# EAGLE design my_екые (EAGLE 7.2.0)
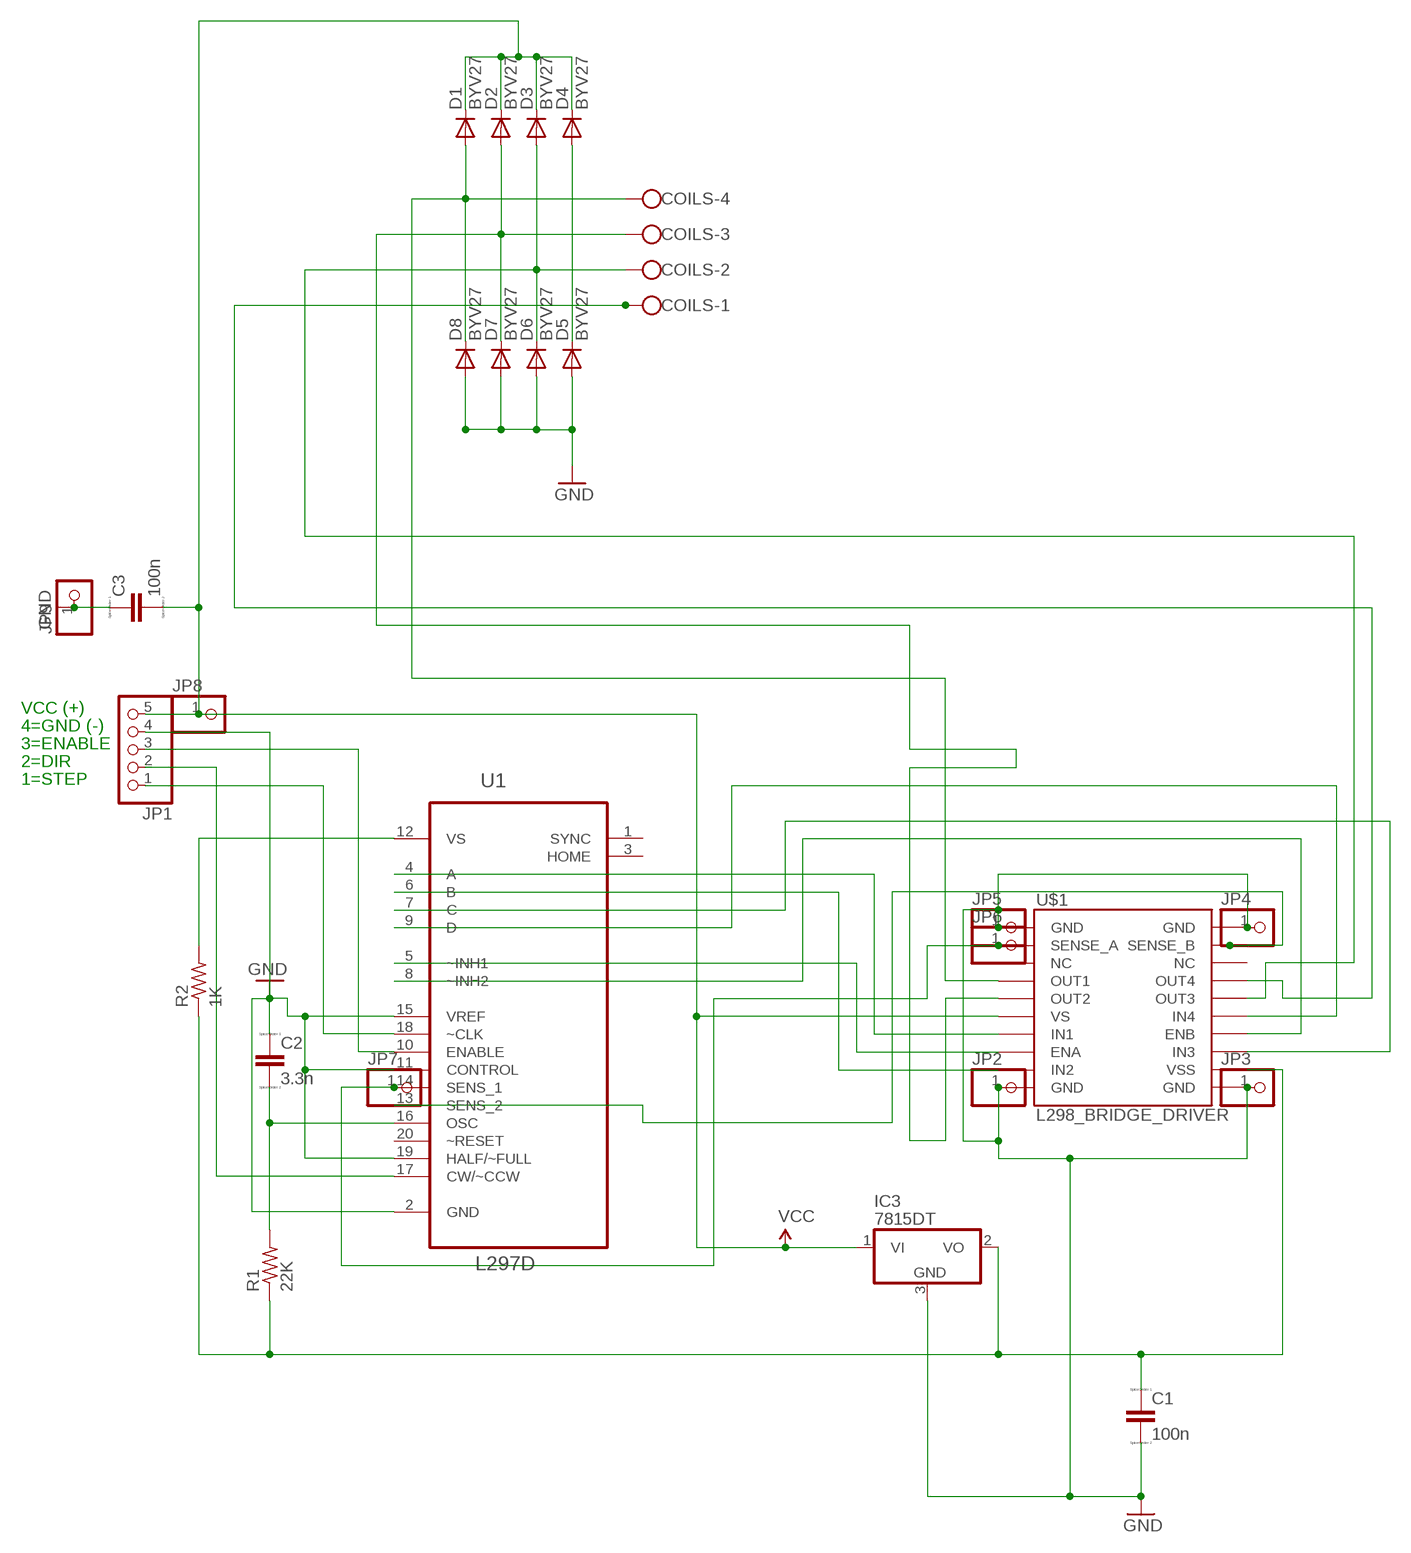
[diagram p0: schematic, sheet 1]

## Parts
C1  100n  CC1206  [C1206]
C2  3.3n  CC1206  [C1206]
C3  100n  CC1206  [C1206]
COILS  W237-4  [W237-4]
D1  BYV27  [SOD57-10]
D2  BYV27  [SOD57-10]
D3  BYV27  [SOD57-10]
D4  BYV27  [SOD57-10]
D5  BYV27  [SOD57-10]
D6  BYV27  [SOD57-10]
D7  BYV27  [SOD57-10]
D8  BYV27  [SOD57-10]
IC3  7815DT  [TO252]
JP1  PINHD-1X55X2MM  [1_05X2MM]
JP2  PINHD-1X1  [1X01]
JP3  PINHD-1X1  [1X01]
JP4  PINHD-1X1  [1X01]
JP5  PINHD-1X1  [1X01]
JP6  PINHD-1X1  [1X01]
JP7  PINHD-1X1  [1X01]
JP8  PINHD-1X1  [1X01]
JP9  PINHD-1X1  [1X01]
R1  22K  RES-US1206  [R1206]
R2  1K  RES-US1206  [R1206]
U1  L297D  [SOIC127P1032X265-20N]
U$1  L298_BRIDGE_DRIVER  [POWERSO20]

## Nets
GND: C1.2 C2.1 C3.1 D5.A D6.A D7.A D8.A IC3.3(GND) JP1.4 JP2.1 JP3.1 JP4.1 JP5.1 JP9.1 U1.2(GND) U1.11(CONTROL) U1.15(VREF) U1.19(HALF/~FULL) U$1.1(GND) U$1.10(GND) U$1.11(GND) U$1.20(GND)
N$1: C1.1 IC3.2(VO) R1.1 R2.1 U$1.12(VSS)
N$2: C2.2 R1.2 U1.16(OSC)
N$3: U1.4(A) U$1.7(IN1)
N$4: U1.6(B) U$1.9(IN2)
N$5: U1.7(C) U$1.13(IN3)
N$6: U1.9(D) U$1.15(IN4)
N$7: U1.5(~INH1) U$1.8(ENA)
N$8: U1.8(~INH2) U$1.14(ENB)
N$9: COILS.4 D1.A D8.C U$1.4(OUT1)
N$10: COILS.3 D2.A D7.C U$1.5(OUT2)
N$11: COILS.2 D3.A D6.C U$1.16(OUT3)
N$12: COILS.1 D4.A D5.C U$1.17(OUT4)
N$13: JP1.1 U1.18(~CLK)
N$14: JP1.3 U1.10(ENABLE)
N$16: JP6.1 JP7.1 U1.14(SENS_1) U$1.2(SENSE_A)
N$17: U1.13(SENS_2) U$1.19(SENSE_B)
N$18: JP1.2 U1.17(CW/~CCW)
N$25: R2.2 U1.12(VS)
VCC: C3.2 D1.C D2.C D3.C D4.C IC3.1(VI) JP1.5 JP8.1 U$1.6(VS)
Unconnected: U1.1(SYNC) U1.3(HOME) U1.20(~RESET) U$1.3(NC) U$1.18(NC)

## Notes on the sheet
- VCC (+)
- 4=GND (-)
- 3=ENABLE
- 2=DIR
- 1=STEP

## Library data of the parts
C1-C3 = eagle-ltspice:C: CAPACITOR, European symbol; SPICEMODEL: NONE; SPICEPREFIX: C
COILS = con-wago-500:W237-4: WAGO SCREW CLAMP
D1-D8 = diode:BYV27: DIODE
IC3 = linear:78*: Positive VOLTAGE REGULATOR Source: http://cache.national.com/ds/LM/LM78L05.pdf http://www.fairchildsemi.com/ds/LM/LM7805.pdf
JP1 = pinhead:PINHD-1X5: PIN HEADER
JP2-JP9 = pinhead:PINHD-1X1: PIN HEADER
R1 R2 = fab:RES-US: Resistor (US Symbol)
U1 = ST Microelctronics_By_element14_Batch_1:L297D: STEPPER MOTOR CONTROLLERS; MPN: L297D; OC_FARNELL: 1467714; OC_NEWARK: 89K0738; PACKAGE: SOICW-20; SUPPLIER: STMICROELECTRONICS
U$1 = SparkFun-PowerIC:L298_BRIDGE_DRIVER: Full-bridge power driver IC

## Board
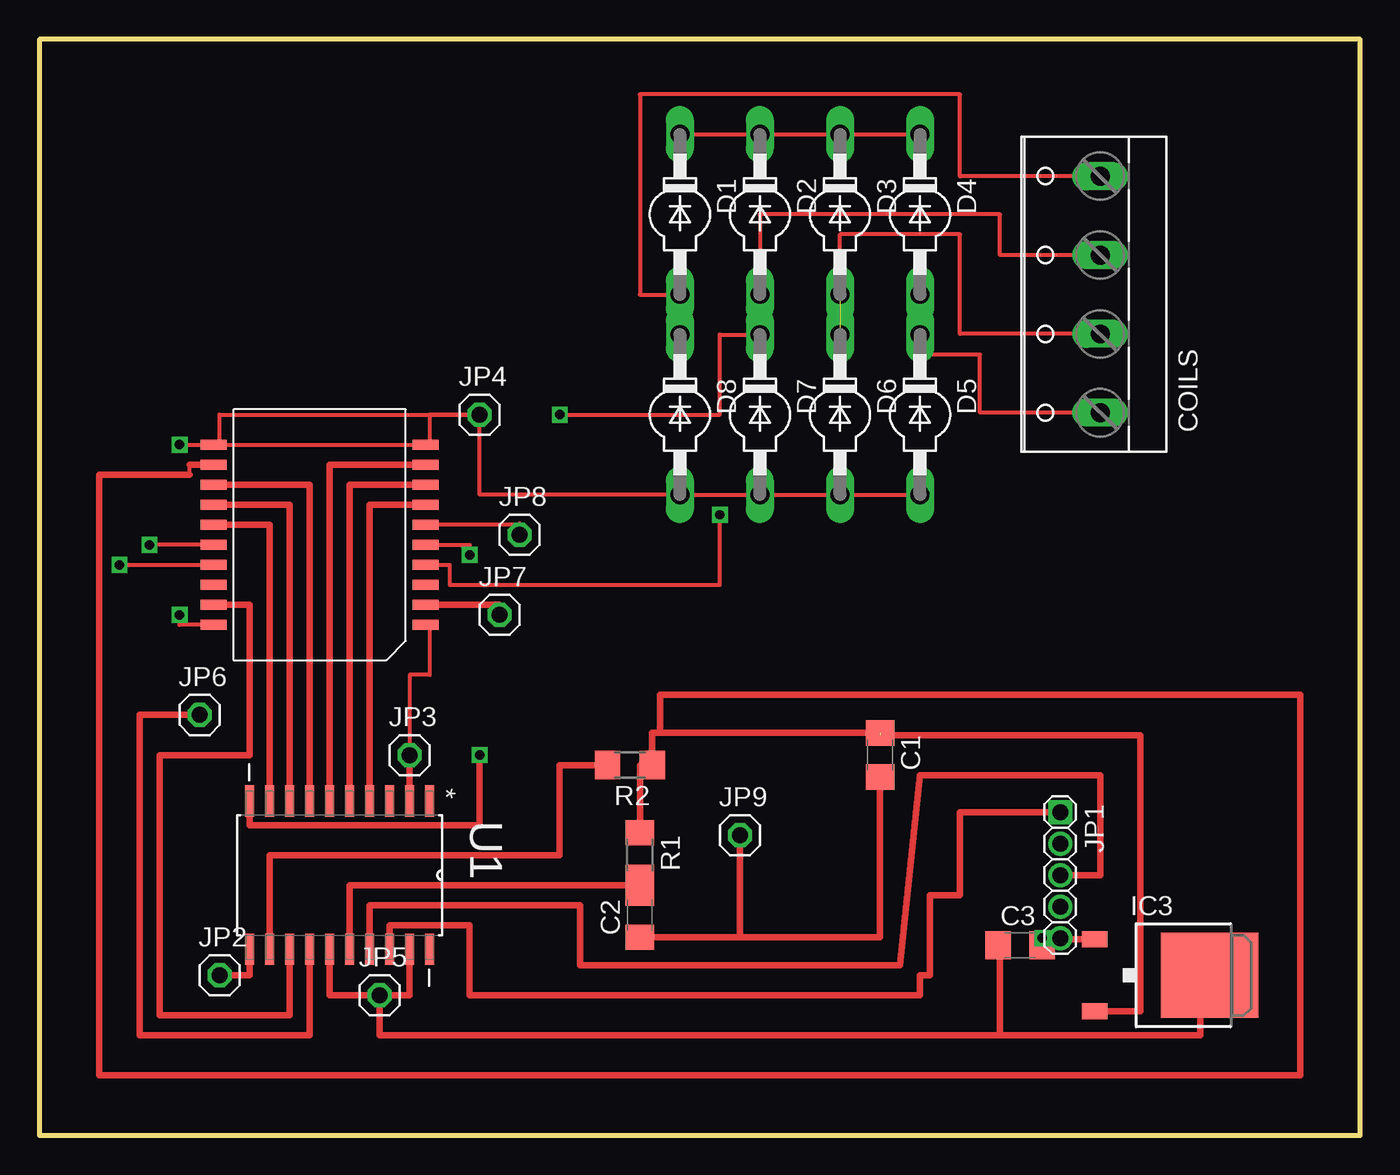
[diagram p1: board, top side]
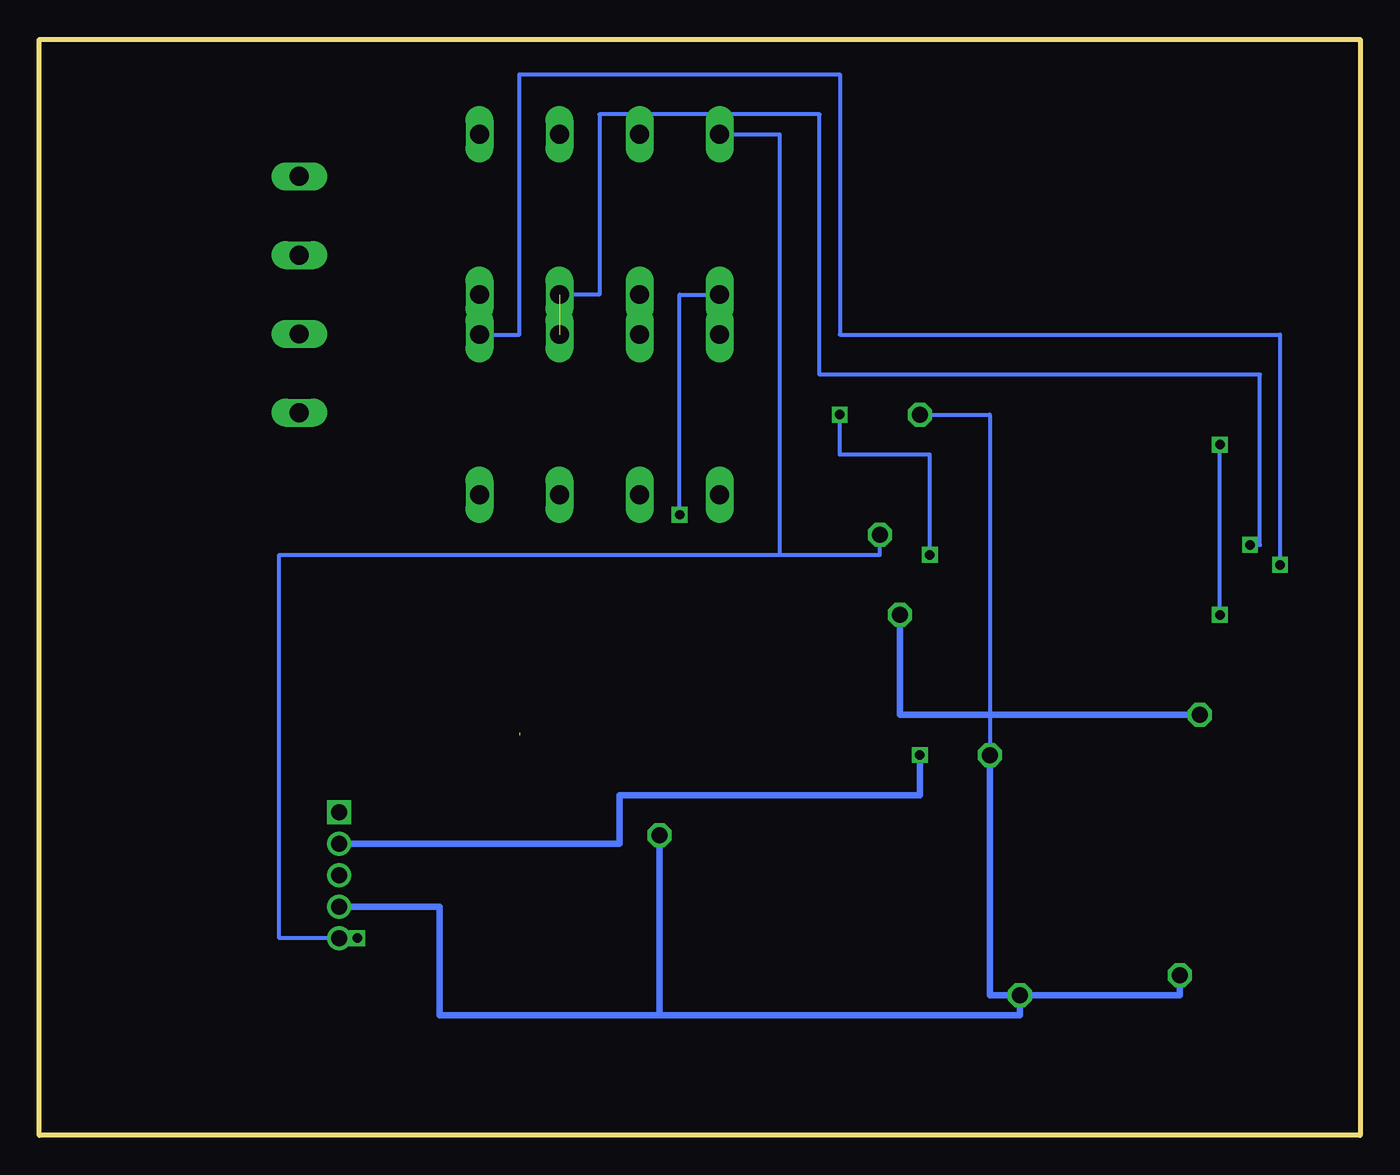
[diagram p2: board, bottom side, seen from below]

Size 83.8 x 69.52 mm. Coordinates in mm from the lower left corner, seen from the top.
Outline: 0,0 83.8,0 83.8,69.52 0,69.52 0,0
Copper layers (1*16): Top 0.035mm / dielectric 1.5mm / Bottom 0.035mm
Design rules "default": minimum track width 10mil, minimum drill 24mil, track to track 8mil, track to pad 8mil, pad to pad 8mil, via to via 8mil, smd to smd 8mil, copper to edge 40mil, drill to drill 8mil, minimum pad ring 10mil, minimum via ring 8mil, stop-mask expansion 4mil, vias tented up to drill 0mil, thermal gap 10mil

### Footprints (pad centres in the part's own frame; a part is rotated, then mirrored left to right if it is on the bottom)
C1206 = smd 1.6 x 1.8: 1 -1.4,0; 2 1.4,0
W237-4 = drill 1.194 long: 1 -7.5,-1.27; 2 -2.5,-1.27; 3 2.5,-1.27; 4 7.5,-1.27
SOD57-10 = drill 1.194 long: A 5.08,0; C -5.08,0
TO252 = smd 1 x 1.6: 1 -2.28,-4.8; 2 2.28,-4.8 | smd 5.4 x 6.2: 3 0,2.5
1_05X2MM = drill 1.016 pad 1.3 square: 1 -4,0 | drill 1.016 pad 1.3: 2 0,0; 3 -2,0; 4 2,0; 5 4,0
1X01 = drill 1.016 octagon: 1 0,0
R1206 = smd 1.6 x 1.803: 1 -1.422,0; 2 1.422,0
SOIC127P1032X265-20N = smd 1.981 x 0.559: 1 -4.699,5.715; 2 -4.699,4.445; 3 -4.699,3.175; 4 -4.699,1.905; 5 -4.699,0.635; 6 -4.699,-0.635; 7 -4.699,-1.905; 8 -4.699,-3.175; 9 -4.699,-4.445; 10 -4.699,-5.715; 11 4.699,-5.715; 12 4.699,-4.445; 13 4.699,-3.175; 14 4.699,-1.905; 15 4.699,-0.635; 16 4.699,0.635; 17 4.699,1.905; 18 4.699,3.175; 19 4.699,4.445; 20 4.699,5.715
POWERSO20 = smd 1.651 x 0.635: 1 -6.731,5.715; 2 -6.731,4.445; 3 -6.731,3.175; 4 -6.731,1.905; 5 -6.731,0.635; 6 -6.731,-0.635; 7 -6.731,-1.905; 8 -6.731,-3.175; 9 -6.731,-4.445; 10 -6.731,-5.715; 11 6.731,-5.715; 12 6.731,-4.445; 13 6.731,-3.175; 14 6.731,-1.905; 15 6.731,-0.635; 16 6.731,0.635; 17 6.731,1.905; 18 6.731,3.175; 19 6.731,4.445; 20 6.731,5.715

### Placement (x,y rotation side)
C1  53.34,24.13 270 top
C2  38.1,13.97 90 top
C3  62.23,12.06 0 top
COILS  66.04,53.34 90 top
D1  40.64,58.42 270 top
D2  45.72,58.42 270 top
D3  50.8,58.42 270 top
D4  55.88,58.42 270 top
D5  55.88,45.72 270 top
D6  50.8,45.72 270 top
D7  45.72,45.72 270 top
D8  40.64,45.72 270 top
IC3  71.75,10.16 270 top
JP1  64.77,16.51 270 top
JP2  11.43,10.16 0 top
JP3  23.5,24.13 0 top
JP4  27.94,45.72 0 top
JP5  21.59,8.89 0 top
JP6  10.16,26.67 0 top
JP7  29.21,33.02 0 top
JP8  30.48,38.1 0 top
JP9  44.45,19.05 0 top
R1  38.1,17.78 270 top
R2  37.46,23.49 180 top
U1  19.05,16.51 270 top
U$1  17.78,38.1 180 top

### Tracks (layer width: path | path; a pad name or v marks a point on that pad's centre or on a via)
GND  (via drill 0.6)
  Top 0.254: 11.43,43.81 U$1.10 | 11.43,43.81 U$1.11 v8.89,43.81 | U$1.20 8.89,32.38 v8.89,33.02 | 11.43,43.81 11.43,45.72 JP4.1 | JP4.1 24.76,45.72 24.76,43.81 | U$1.1 24.76,32.38 24.76,29.21 23.5,29.21 JP3.1 | D5.A D6.A D7.A D8.A 27.94,40.64 JP4.1
  Top 0.406: JP2.1 13.33,10.16 U1.11 | U1.19 23.5,8.89 JP5.1 | JP5.1 18.42,8.89 U1.15 | U1.2 JP3.1 | C2.1 44.45,12.57 | C1.2 53.34,12.57 44.45,12.57 | C3.1 60.96,12.06 60.96,6.35 | 60.96,6.35 21.59,6.35 JP5.1 | IC3.3 73.66,10.16 73.66,6.35 60.96,6.35 | 44.45,12.57 JP9.1
  Bottom 0.254: v8.89,33.02 v8.89,43.81 | JP4.1 23.5,45.72 JP3.1
  Bottom 0.406: JP5.1 11.43,8.89 JP2.1 | JP3.1 23.5,8.89 JP5.1 | JP1.4 58.42,14.51 58.42,7.62 44.45,7.62 | 44.45,7.62 21.59,7.62 JP5.1 | JP9.1 44.45,7.62
  other vias: 27.94,45.72
N$1  (1 unrouted)
  Top 0.254: 9.53,41.91 9.53,42.55
  Top 0.406: IC3.2 69.85,7.88 69.85,25.4 53.34,25.4 | C1.1 39.37,25.53 | R1.1 38.1,23.49 R2.1 38.89,25.53 39.37,25.53 | 39.37,25.53 39.37,27.94 80.01,27.94 80.01,3.81 3.81,3.81 3.81,41.91 9.53,41.91 | 9.53,42.55 U$1.12
N$2
  Top 0.406: U1.16 19.68,15.88 38.1,15.88 C2.2 R1.2
N$3
  Top 0.406: U1.4 20.96,40 U$1.7
N$4
  Top 0.406: U1.6 18.42,42.55 U$1.9
N$5
  Top 0.406: U1.7 17.14,41.27 U$1.13
N$6
  Top 0.406: U1.9 14.61,38.73 U$1.15
N$7
  Top 0.406: U1.5 19.68,41.27 U$1.8
N$8
  Top 0.406: U1.8 15.87,40 U$1.14
N$9  (via drill 0.6)
  Top 0.254: COILS.4 58.42,60.84 58.42,66.04 38.1,66.04 38.1,53.34 D1.A D8.C | U$1.4 26.04,36.2 26.04,34.92 43.18,34.92 v43.18,39.37
  Bottom 0.254: v43.18,39.37 43.18,53.34 D1.A
N$10  (via drill 0.6)
  Top 0.254: COILS.3 60.96,55.84 60.96,58.42 45.72,58.42 D2.A D7.C 43.18,50.8 43.18,45.72 v33.02,45.72 | U$1.5 27.3,37.46 v27.3,36.83
  Bottom 0.254: v27.3,36.83 27.3,43.18 33.02,43.18 v33.02,45.72
N$11  (via drill 0.6)  (1 unrouted)
  Top 0.254: COILS.2 58.42,50.84 58.42,57.15 50.8,57.15 D6.C | U$1.16 v6.99,37.46
  Bottom 0.254: v6.99,37.46 6.35,37.46 6.35,48.26 34.29,48.26 34.29,64.77 48.26,64.77 48.26,53.34 D3.A
N$12  (via drill 0.6)
  Top 0.254: COILS.1 59.69,45.84 59.69,49.53 55.88,49.53 D5.C D4.A | v5.08,36.2 U$1.17
  Bottom 0.254: D5.C 53.34,50.8 53.34,67.31 33.02,67.31 33.02,50.8 5.08,50.8 v5.08,36.2
N$13
  Top 0.406: JP1.1 58.42,20.51 58.42,15.24 56.52,15.24 56.52,10.16 55.88,10.16 55.88,8.89 27.3,8.89 27.3,13.34 22.22,13.34 U1.18
N$14  (via drill 0.6)
  Top 0.406: U1.10 13.33,19.68 27.94,19.68 v27.94,24.13
  Bottom 0.406: JP1.3 46.99,18.51 46.99,21.59 27.94,21.59 v27.94,24.13
N$16
  Top 0.406: U$1.2 29.21,33.66 JP7.1 | U1.14 17.14,6.35 6.35,6.35 6.35,26.67 JP6.1
  Bottom 0.406: JP6.1 29.21,26.67 JP7.1
N$17
  Top 0.406: U1.13 15.87,7.62 7.62,7.62 7.62,24.13 13.33,24.13 13.33,33.66 U$1.19
N$18
  Top 0.406: U1.17 20.96,14.61 34.29,14.61 34.29,10.8 54.61,10.8 55.88,22.86 67.31,22.86 67.31,16.51 JP1.2
N$25
  Top 0.406: U1.12 14.61,17.78 33.02,17.78 33.02,23.49 R2.2
VCC  (via drill 0.6)
  Top 0.254: 30.48,38.73 U$1.6 | D1.C D2.C D3.C D4.C
  Top 0.406: C3.2 v63.63,12.51 JP1.5 64.77,12.44 IC3.1 | 30.48,38.73 JP8.1
  Bottom 0.254: v63.63,12.51 68.58,12.51 68.58,36.83 36.83,36.83 | 36.83,36.83 30.48,36.83 JP8.1 | D1.C 36.83,63.5 36.83,36.83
